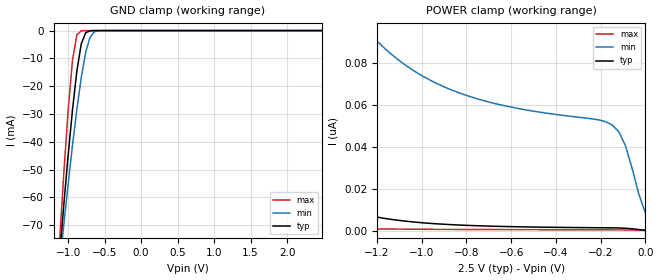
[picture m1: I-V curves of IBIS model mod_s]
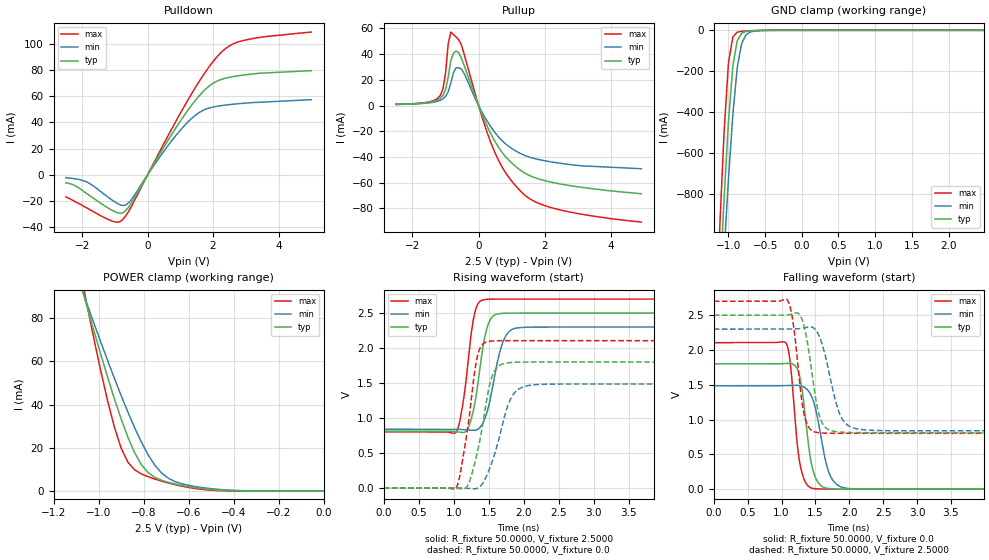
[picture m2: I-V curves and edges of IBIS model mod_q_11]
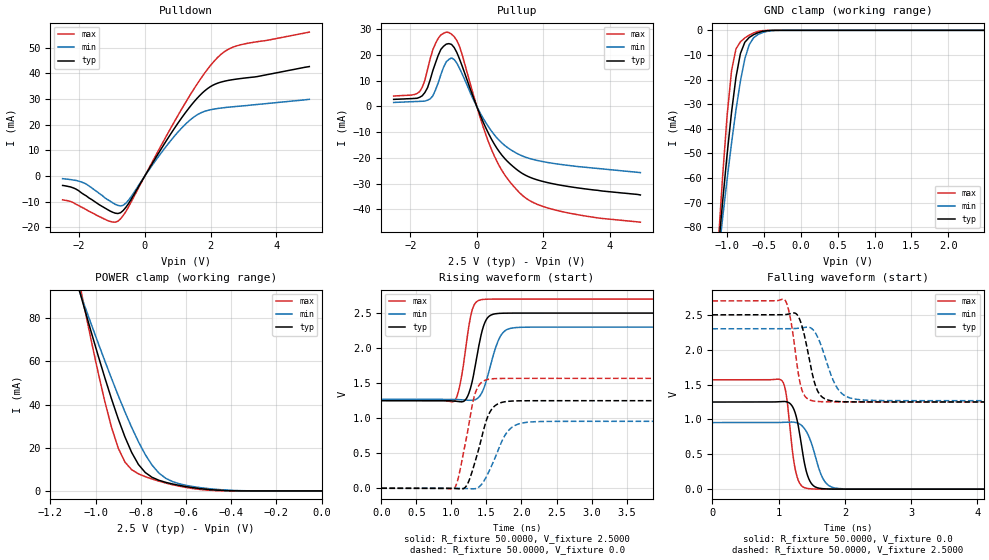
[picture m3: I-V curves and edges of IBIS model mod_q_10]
| IBIS (I/O, Buffer, Information, Specification) Model, officially
| electronic behavioral standard for Buffer structures of digital pins.
[IBIS ver]  4.0
[File name] pe_22_m95p32_2d5.ibs
[File Rev]  1.0
[Date]   12 Dec 2024
[Source]   CAD & Design Services (Catania) - STMicroelectronics
[Notes]
   (Note1)  This IBIS model includes the SO8N package parasitic data
   (Note2)  Pin 2 (S) and Pin 3,5,7 (WO2,DO0,HO3) have four driver
   stength cases: High, Medium, Qlow, Low;
   (Note3)  This IBIS model has some Notes about the non-monotonicity
   of the I-V curves, but they are not indicative of problems
   inside the model;
[Disclaimer]
   Customers are solely responsible for all aspects of their
   own product designs or applications using this IBIS Model.
   STMicroelectronics assumes no liability for Custmer Designs
   and applications associated to this IBIS Model.
   In the use of this IBIS Model Customer shall not modify,
   disassemble, alter this Model in whole or in part.
   If Customers do not accept these terms, the IBIS Model
   may not be used. For any problems or modifications please
   contact STMicroelectronics (www.st.com).
[Copyright] (c) 2024 STMicroelectronics
|   Component M95P32
[Component] M95P32
[Manufacturer] STMicroelectronics
[Package]
| variable   typ   min   max
R_pkg   0.0   0.0   0.0
L_pkg   0.0H   0.0H   0.0H
C_pkg   0.0F   0.0F   0.0F
[Pin]  signal_name   model_name   R_pin   L_pin   C_pin
1   S   mod_s   129.1m   2.1741nH   1.0266pF
2   QO1   mod_q   89.7m   1.6160nH   0.3359pF
3   WO2   mod_dwh   91.2m   1.6289nH   0.3576pF
4   VSS   GND   130.9m   2.1824nH   0.2874pF
5   DO0   mod_dwh   130.7m   2.1818nH   0.2862pF
6   C   mod_c   85.3m   1.5892nH   0.3544pF
7   HO3   mod_dwh   84.5m   1.5827nH   0.3547pF
8   VDD   POWER   124.1m   2.1422nH   0.2841pF
[Model Selector]   mod_q
mod_q_11   High drive: bit0='1', bit1='1'
mod_q_10   Med drive:  bit0='1', bit1='0'
mod_q_01   Qlow drive: bit0='0', bit1='1'
mod_q_00   Low drive:  bit0='0', bit1='0'
[Model Selector]   mod_dwh
mod_dwh_11   High drive: bit0='1', bit1='1'
mod_dwh_10   Med drive:  bit0='1', bit1='0'
mod_dwh_01   Qlow drive: bit0='0', bit1='1'
mod_dwh_00   Low drive:  bit0='0', bit1='0'
| Models and submodels in the file (10): mod_s (Input), mod_q_11 (Output), mod_q_10 (Output), mod_q_01 (Output), mod_q_00 (Output), mod_c (Input), mod_dwh_11 (I/O), mod_dwh_10 (I/O), mod_dwh_01 (I/O), mod_dwh_00 (I/O)
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|   Model mod_s
[Model]   mod_s
Model_type Input
Vinl   =   0.540V
Vinh   =   1.260V
C_comp   1.014pF   0.968pF   1.062pF
[Model Spec]
Vinl   0.750V  0.690V  0.810V  | <- for Vcc = 2.5V, 2.3V, 2.7V
Vinh   1.750V  1.610V  1.890V  | <- for Vcc = 2.5V, 2.3V, 2.7V
[Temperature Range]  25.0000   0.1050k   -40.0000
[Voltage Range]   2.5000V   2.3000V   2.7000V
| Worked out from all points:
|   GND clamp passes 1 mA (typ) near -0.76 V on its own axis
[GND_clamp]
|Voltage   I(typ)   I(min)   I(max)
-2.5V     -572.7mA   -475mA     -759.1mA
-1.12V    -81.87mA   -85.46mA   -77.2mA
-1.06V    -62.91mA   -70.12mA   -51.71mA
-1V       -44.93mA   -55.32mA   -28.75mA
-940mV    -28.48mA   -41.26mA   -10.62mA
-880mV    -14.54mA   -28.26mA   -1.54mA
-820mV    -4.805mA   -16.86mA   -92.72uA
-760mV    -792.9uA   -7.883mA   -4.745uA
-700mV    -84.66uA   -2.422mA   -241.6nA
-640mV    -8.294uA   -462.2uA   -12.61nA
-580mV    -804.9nA   -70.25uA   -745.3pA
2.48V     143.4pA    51.97nA    21.5pA
[POWER_clamp]
|Voltage   I(typ)   I(min)   I(max)
-2.49V    390.7nA    883.4nA    118.4nA
-2.43V    336.6nA    797.5nA    94.45nA
-2.22V    190.6nA    547.7nA    39.52nA
-2.01V    100.3nA    367.4nA    15.01nA
-1.89V    67.45nA    290.7nA    8.517nA
-1.65V    29.21nA    183nA      2.957nA
-1.35V    10.35nA    110.3nA    1.146nA
-1.23V    7.081nA    93.69nA    908.9pA
-810mV    2.603nA    64.74nA    599.3pA
-150mV    1.351nA    50.46nA    408.5pA
-90mV     1.173nA    40.65nA    372.5pA
0V        258.1pA    8.425nA    117.7pA
|   Model mod_q_11
[Model]   mod_q_11
Model_type Output
Polarity   Non-Inverting
Enable   Active-High
Vmeas  =   1.250V
Cref   =   30pF
C_comp   1.466pF   1.400pF   1.535pF
[Model Spec]
Vmeas  1.250V  1.150V  1.350V  | <- for Vcc = 2.5V, 2.3V, 2.7V
[Temperature Range]  25.0000   0.1050k   -40.0000
[Voltage Range]   2.5000V   2.3000V   2.7000V
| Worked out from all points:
|   slope of the pulldown table from 0 to 0.375 V, typ, clamps not added: 23.4 ohm
|   slope of the pullup table from 0 to 0.375 V, typ, clamps not added: 16.9 ohm
|   GND clamp passes 1 mA (typ) near -0.58 V on its own axis
|   POWER clamp passes 1 mA (typ) near -0.53 V on its own axis
|   rising waveform, R_fixture 50.0000, V_fixture 2.5000: 20-80 % time 156ps typ, 187ps min, 139ps max; typ from 0.812 V to 2.5 V
|   rising waveform, R_fixture 50.0000, V_fixture 0.0: 20-80 % time 205ps typ, 257ps min, 172ps max; typ from 0 V to 1.8 V
|   falling waveform, R_fixture 50.0000, V_fixture 0.0: 20-80 % time 141ps typ, 187ps min, 119ps max; typ from 1.8 V to 0 V
|   falling waveform, R_fixture 50.0000, V_fixture 2.5000: 20-80 % time 162ps typ, 218ps min, 132ps max; typ from 2.5 V to 0.812 V
[Pulldown]
|Voltage   I(typ)   I(min)   I(max)
-2.5V     -6.1mA     -2.16mA    -16.8mA
-1.86V    -14.3mA    -5.4mA     -25.2mA
-1.14V    -26.3mA    -18.3mA    -34.7mA
-820mV    -29.37mA   -23.05mA   -35.38mA
-660mV    -27.05mA   -22.93mA   -30.99mA
-500mV    -21.73mA   -19.06mA   -24.39mA
540mV     22.88mA    19.46mA    25.84mA
1.26V     50.29mA    41.01mA    58.29mA
1.74V     64.59mA    49.68mA    77.47mA
2.22V     72.5mA     52.68mA    92.69mA
2.94V     76.14mA    54.59mA    102.6mA
5V        79.45mA    57.32mA    108.9mA
[Pullup]
|Voltage   I(typ)   I(min)   I(max)
-2.5V     960uA      860uA      1.01mA
-1.16V    5.71mA     4.1mA      7.9mA
-1V       12.31mA    7.124mA    25.18mA
-920mV    22.01mA    10.66mA    47.97mA
-840mV    35.12mA    17.46mA    57.19mA
-680mV    42.55mA    29.43mA    53.34mA
-520mV    36.76mA    28.49mA    47.15mA
440mV     -25.32mA   -19.07mA   -33.28mA
840mV     -40.44mA   -30.28mA   -53.17mA
1.32V     -51.25mA   -37.92mA   -67.9mA
2.36V     -60.43mA   -44.46mA   -80.5mA
4.92V     -68.6mA    -49.1mA    -90.7mA
[GND_clamp]
|Voltage   I(typ)   I(min)   I(max)
-2.5V     -12.69A    -11.53A    -14.4A
-1.12V    -1.259A    -1.484A    -977mA
-1.06V    -828.4mA   -1.093A    -501.9mA
-1V       -448.3mA   -729mA     -159.9mA
-940mV    -174mA     -412mA     -32.51mA
-880mV    -50.2mA    -181.6mA   -8.897mA
-820mV    -14.26mA   -64.74mA   -4.945mA
-760mV    -5.535mA   -21.85mA   -3.213mA
-700mV    -3.068mA   -7.635mA   -1.989mA
-640mV    -1.821mA   -3.347mA   -1.073mA
-340mV    -4.191uA   -40.02uA   -134.6nA
2.48V     343.3pA    931.5nA    131.5pA
[POWER_clamp]
|Voltage   I(typ)   I(min)   I(max)
-2.49V    667.2mA    541mA      921mA
-1.08V    96.07mA    95.11mA    101.2mA
-1.05V    84.91mA    86.28mA    85.45mA
-990mV    63.23mA    68.98mA    55.57mA
-930mV    42.88mA    52.31mA    29.76mA
-900mV    33.53mA    44.31mA    19.96mA
-840mV    17.8mA     29.4mA     9.816mA
-810mV    12.22mA    22.72mA    7.905mA
-750mV    6.305mA    11.96mA    5.516mA
-660mV    3.226mA    4.34mA     2.89mA
-420mV    154.8uA    392.4uA    29.01uA
0V        492.2pA    14.11nA    240.5pA
[Ramp]
| variable   typ   min   max
dV/dt_r  1.0800/0.2734n   0.9088/0.3125n   1.2634/0.2481n
dV/dt_f  1.0131/0.2548n   0.8870/0.2879n   1.1391/0.2416n
R_load = 50.0000
[Rising Waveform]
R_fixture= 50.0000
V_fixture= 2.5000
V_fixture_min= 2.3000
V_fixture_max= 2.7000
|time   V(typ)   V(min)   V(max)
0s        811.6mV    838.9mV    801.5mV
1.032ns   805.5mV    838.8mV    791.4mV
1.136ns   792.6mV    833.7mV    1.232V
1.24ns    946.3mV    825.7mV    2.12V
1.32ns    1.314V     828.4mV    2.569V
1.432ns   2.093V     959.8mV    2.691V
1.528ns   2.415V     1.297V     2.699V
1.688ns   2.495V     2.043V     2.7V
1.896ns   2.5V       2.285V     2.7V
8ns       2.5V       2.3V       2.7V
[Rising Waveform]
R_fixture= 50.0000
V_fixture= 0.0
V_fixture_min= 0.0
V_fixture_max= 0.0
|time   V(typ)   V(min)   V(max)
0s        3.45nV     419.9nV    574.2pV
1.024ns   -2.38mV    831.1uV    -11.17mV
1.096ns   -9.776mV   -3.697uV   217.3mV
1.24ns    135.2mV    -7.605mV   1.162V
1.352ns   575.4mV    1.858mV    1.935V
1.48ns    1.31V      196.2mV    2.091V
1.592ns   1.688V     506.4mV    2.104V
1.8ns     1.792V     1.244V     2.106V
2.056ns   1.8V       1.462V     2.106V
8ns       1.8V       1.486V     2.106V
[Falling Waveform]
R_fixture= 50.0000
V_fixture= 0.0
V_fixture_min= 0.0
V_fixture_max= 0.0
|time   V(typ)   V(min)   V(max)
0s        1.8V       1.486V     2.106V
1.064ns   1.807V     1.488V     2.101V
1.128ns   1.805V     1.491V     1.823V
1.224ns   1.745V     1.493V     720.8mV
1.272ns   1.603V     1.487V     361.8mV
1.448ns   334.1mV    1.322V     13.96mV
1.544ns   91.4mV     959.1mV    3.748mV
1.688ns   9.787mV    270.8mV    674.4uV
1.928ns   1.005mV    17.9mV     42.02uV
8ns       962.7nV    1.54uV     983.6nV
[Falling Waveform]
R_fixture= 50.0000
V_fixture= 2.5000
V_fixture_min= 2.3000
V_fixture_max= 2.7000
|time   V(typ)   V(min)   V(max)
0s        2.5V       2.3V       2.7V
1.088ns   2.504V     2.299V     2.717V
1.176ns   2.523V     2.301V     2.356V
1.304ns   2.434V     2.312V     1.234V
1.384ns   2.095V     2.327V     920.6mV
1.496ns   1.347V     2.298V     820.1mV
1.608ns   938mV      2.053V     806.5mV
1.848ns   821.6mV    1.107V     801.8mV
2.088ns   812.9mV    872mV      801.5mV
8ns       811.6mV    838.9mV    801.5mV
|   Model mod_q_10
[Model]   mod_q_10
Model_type Output
Polarity   Non-Inverting
Enable   Active-High
Vmeas  =   1.250V
Cref   =   30pF
C_comp   1.466pF   1.400pF   1.535pF
[Model Spec]
Vmeas  1.250V  1.150V  1.350V  | <- for Vcc = 2.5V, 2.3V, 2.7V
[Temperature Range]  25.0000   0.1050k   -40.0000
[Voltage Range]   2.5000V   2.3000V   2.7000V
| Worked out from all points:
|   slope of the pulldown table from 0 to 0.375 V, typ, clamps not added: 46.8 ohm
|   slope of the pullup table from 0 to 0.375 V, typ, clamps not added: 33.9 ohm
|   GND clamp passes 1 mA (typ) near -0.58 V on its own axis
|   POWER clamp passes 1 mA (typ) near -0.53 V on its own axis
|   rising waveform, R_fixture 50.0000, V_fixture 2.5000: 20-80 % time 148ps typ, 183ps min, 131ps max; typ from 1.25 V to 2.5 V
|   rising waveform, R_fixture 50.0000, V_fixture 0.0: 20-80 % time 210ps typ, 257ps min, 178ps max; typ from 0 V to 1.25 V
|   falling waveform, R_fixture 50.0000, V_fixture 0.0: 20-80 % time 144ps typ, 197ps min, 116ps max; typ from 1.25 V to 0 V
|   falling waveform, R_fixture 50.0000, V_fixture 2.5000: 20-80 % time 173ps typ, 240ps min, 135ps max; typ from 2.5 V to 1.25 V
[Pulldown]
|Voltage   I(typ)   I(min)   I(max)
-2.5V     -3.72mA    -1.07mA    -9.34mA
-1.86V    -7.2mA     -2.7mA     -12.6mA
-1.14V    -13.1mA    -9.2mA     -17.4mA
-820mV    -14.69mA   -11.52mA   -17.69mA
-660mV    -13.52mA   -11.47mA   -15.5mA
-500mV    -10.87mA   -9.532mA   -12.19mA
540mV     11.44mA    9.728mA    12.92mA
1.26V     25.15mA    20.5mA     29.15mA
1.74V     32.3mA     24.84mA    38.73mA
2.22V     36.25mA    26.34mA    46.35mA
2.86V     37.94mA    27.21mA    51.03mA
5V        42.7mA     29.9mA     56.16mA
[Pullup]
|Voltage   I(typ)   I(min)   I(max)
-2.5V     2.762mA    1.562mA    4.052mA
-1.72V    3.553mA    1.982mA    5.743mA
-1.48V    7.344mA    2.457mA    14.39mA
-1.24V    16.99mA    6.442mA    24.51mA
-1.08V    22.2mA     12.4mA     27.82mA
-840mV    24.44mA    18.28mA    28.74mA
-520mV    18.48mA    14.85mA    23.37mA
120mV     -3.865mA   -2.929mA   -5.077mA
520mV     -14.48mA   -10.9mA    -19.03mA
1.32V     -25.62mA   -18.96mA   -33.95mA
2.44V     -30.41mA   -22.38mA   -40.5mA
4.92V     -34.4mA    -25.7mA    -44.98mA
[GND_clamp]
|Voltage   I(typ)   I(min)   I(max)
-2.5V     -618.8mA   -507.1mA   -839.7mA
-1.12V    -89.51mA   -92.19mA   -86.51mA
-1.06V    -69.34mA   -76.02mA   -58.94mA
-1V       -50.38mA   -60.48mA   -34.64mA
-940mV    -33.28mA   -45.81mA   -16.38mA
-880mV    -19.11mA   -32.38mA   -7.564mA
-820mV    -9.453mA   -20.71mA   -4.67mA
-760mV    -4.854mA   -11.6mA    -3.093mA
-700mV    -2.891mA   -5.814mA   -1.933mA
-580mV    -964.2uA   -1.685mA   -447.5uA
-340mV    -4.19uA    -39.9uA    -134.6nA
2.48V     343.3pA    931.5nA    131.5pA
[POWER_clamp]
|Voltage   I(typ)   I(min)   I(max)
-2.49V    667.2mA    541mA      921mA
-1.08V    96.07mA    95.11mA    101.2mA
-1.05V    84.91mA    86.28mA    85.45mA
-990mV    63.23mA    68.98mA    55.57mA
-930mV    42.88mA    52.31mA    29.76mA
-900mV    33.53mA    44.31mA    19.96mA
-840mV    17.8mA     29.4mA     9.816mA
-810mV    12.22mA    22.72mA    7.905mA
-750mV    6.305mA    11.96mA    5.516mA
-660mV    3.226mA    4.34mA     2.89mA
-420mV    154.8uA    392.4uA    29.01uA
0V        492.2pA    14.11nA    240.5pA
[Ramp]
| variable   typ   min   max
dV/dt_r   0.7498/0.2355n   0.5900/0.3071n   0.9410/0.1910n
dV/dt_f   0.7496/0.2142n   0.6311/0.3208n   0.8690/0.1617n
R_load = 50.0000
[Rising Waveform]
R_fixture= 50.0000
V_fixture= 2.5000
V_fixture_min= 2.3000
V_fixture_max= 2.7000
|time   V(typ)   V(min)   V(max)
0s        1.251V     1.269V     1.252V
1.04ns    1.244V     1.268V     1.24V
1.136ns   1.233V     1.263V     1.547V
1.248ns   1.353V     1.256V     2.308V
1.312ns   1.597V     1.257V     2.59V
1.424ns   2.189V     1.345V     2.691V
1.52ns    2.438V     1.611V     2.699V
1.68ns    2.496V     2.132V     2.7V
1.872ns   2.5V       2.288V     2.7V
8ns       2.5V       2.3V       2.7V
[Rising Waveform]
R_fixture= 50.0000
V_fixture= 0.0
V_fixture_min= 0.0
V_fixture_max= 0.0
|time   V(typ)   V(min)   V(max)
0s        5.246nV    623.3nV    889pV
1.04ns    -2.183mV   587.5uV    -1.489mV
1.104ns   -7.264mV   -5.605nV   170.9mV
1.2ns     16.06mV    -2.904mV   644.9mV
1.344ns   399.9mV    -4.835mV   1.369V
1.424ns   692.4mV    48.27mV    1.506V
1.536ns   1.062V     240.9mV    1.556V
1.792ns   1.239V     797.6mV    1.568V
2.08ns    1.249V     941.7mV    1.568V
8ns       1.25V      955.1mV    1.568V
[Falling Waveform]
R_fixture= 50.0000
V_fixture= 0.0
V_fixture_min= 0.0
V_fixture_max= 0.0
|time   V(typ)   V(min)   V(max)
0s        1.25V      955.1mV    1.568V
1.056ns   1.258V     957.9mV    1.549V
1.12ns    1.253V     961.1mV    1.325V
1.216ns   1.173V     962.2mV    490.1mV
1.264ns   1.048V     955.2mV    228.3mV
1.424ns   235.5mV    817.6mV    12.35mV
1.52ns    53.72mV    586.1mV    2.853mV
1.664ns   7.123mV    161.3mV    372.6uV
1.888ns   595.9uV    11.41mV    22.35uV
8ns       1.028uV    1.623uV    1.112uV
[Falling Waveform]
R_fixture= 50.0000
V_fixture= 2.5000
V_fixture_min= 2.3000
V_fixture_max= 2.7000
|time   V(typ)   V(min)   V(max)
0s        2.5V       2.3V       2.7V
1.088ns   2.503V     2.299V     2.72V
1.184ns   2.519V     2.301V     2.418V
1.28ns    2.501V     2.306V     1.77V
1.344ns   2.365V     2.313V     1.447V
1.52ns    1.607V     2.286V     1.265V
1.648ns   1.329V     2.044V     1.254V
1.872ns   1.259V     1.469V     1.252V
2.16ns    1.251V     1.291V     1.252V
8ns       1.251V     1.269V     1.252V
